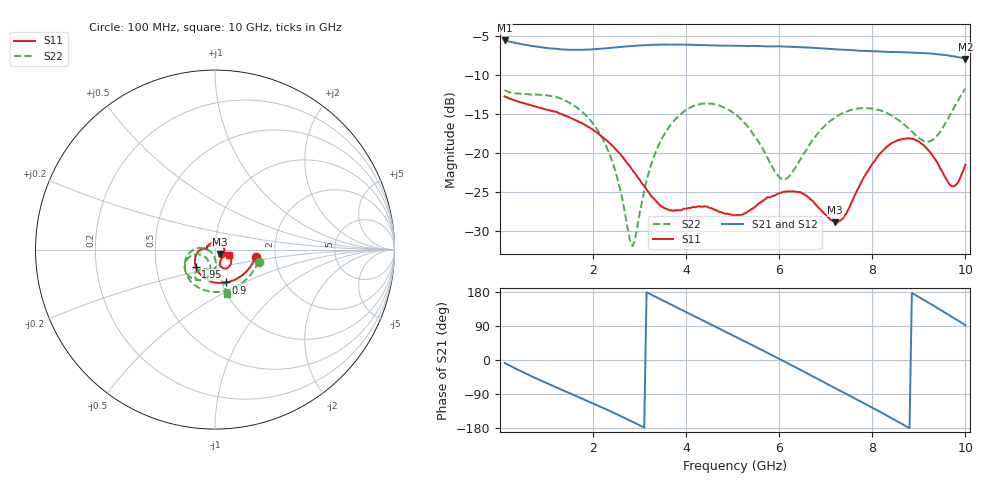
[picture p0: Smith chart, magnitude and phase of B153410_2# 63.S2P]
!  2-Port S-parameters saved by WinCal
! VAR MeasName=S-Parameters (CALIBRATED_DATA) read from VNA (N5245A)
! VAR MeasDate=2016-12-23 10:02:45
! VAR NAME=B153410_2# 63
! VAR FILENAME=B153410_2# 63.S2P
! VAR DATE=2016-12-23 10:02:45
! VAR PHYS_PORTS=1,2
# Hz S DB R 50
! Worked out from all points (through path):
!   199 points, 100 MHz to 10 GHz, reference 50 ohm
!   highest |S21| = -5.60 dB at 100 MHz (marker M1); lowest = -8.0 dB at 10 GHz (marker M2)
!   group delay of S21, straight-line fit = 172 ps
!   lowest |S11| = -28.9 dB at 7.2 GHz (marker M3), VSWR 1.07, Z = 52.6 - j2.59 ohm
!   |S11| at or under -10 dB: start of sweep to end of sweep
!   |S22| runs from -31.9 to -11.8 dB; largest |S21 - S12| = 0.0027
!   S11 on the Smith chart (normalised r, x): 100 MHz: 1.58, -0.15; 900 MHz: 1.06, -0.40; 1.95 GHz: 0.79, -0.16; 10 GHz: 1.17, -0.07
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1e8  -12.76 -11.0  -5.60 -7.8  -5.62 -7.8  -11.98 -15.3
5e8  -13.60 -42.7  -6.11 -32.6  -6.11 -32.5  -12.44 -60.0
9e8  -14.28 -71.1  -6.49 -55.2  -6.49 -55.1  -12.58 -96.7
1.75e9  -16.15 -126.3  -6.80 -101.0  -6.79 -101.0  -14.65 -155.8
1.95e9  -16.85 -138.0  -6.74 -111.7  -6.74 -111.7  -15.87 -166.8
2.45e9  -19.30 -164.9  -6.51 -139.6  -6.50 -139.7  -21.75 173.3
2.85e9  -22.23 179.5  -6.31 -163.1  -6.30 -163.2  -31.95 -134.5
3.15e9  -24.69 173.9  -6.19 178.7  -6.20 178.7  -23.54 -86.6
3.4e9  -26.49 175.3  -6.15 163.4  -6.14 163.4  -19.11 -90.6
3.8e9  -27.32 178.3  -6.12 138.7  -6.13 138.8  -15.50 -106.5
4.25e9  -26.85 164.9  -6.17 111.2  -6.18 111.2  -13.82 -126.4
5.05e9  -27.99 89.4  -6.28 62.3  -6.29 62.5  -15.05 -157.4
5.6e9  -26.33 21.7  -6.32 28.2  -6.32 28.2  -19.03 -166.6
6.05e9  -25.08 -19.9  -6.37 -0.0  -6.38 0.0  -23.35 -141.3
6.7e9  -26.10 -54.3  -6.53 -41.7  -6.54 -41.6  -18.50 -103.1
7.2e9  -28.88 -43.1  -6.72 -73.9  -6.73 -73.7  -15.46 -108.6
7.75e9  -23.90 -17.9  -6.93 -109.4  -6.91 -109.2  -14.28 -119.6
8.35e9  -19.03 -35.7  -7.07 -149.0  -7.05 -148.7  -14.99 -129.1
8.8e9  -18.14 -55.7  -7.15 -179.9  -7.14 -179.6  -16.98 -127.3
9.25e9  -19.99 -71.0  -7.27 148.2  -7.27 148.2  -18.49 -102.2
9.7e9  -24.23 -51.3  -7.61 114.6  -7.60 114.9  -14.82 -77.0
1e10  -21.51 -19.4  -7.95 91.9  -7.99 92.1  -11.76 -75.6
